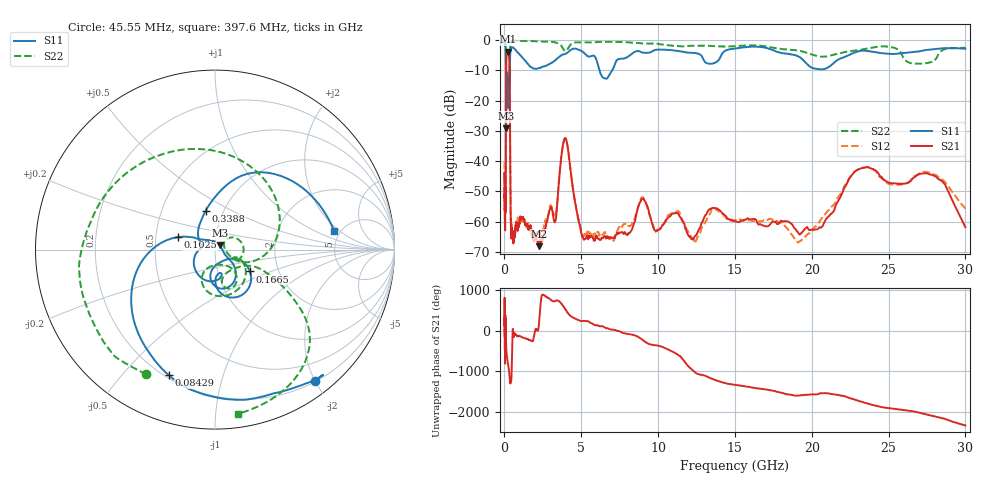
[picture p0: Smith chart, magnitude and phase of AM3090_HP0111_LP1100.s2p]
! Date/Time: Thu, Feb 28, 2019 2:01 PM
! Network Analyzer: Agilent Technologies E8364B Rev: A.07.50.67
! Sweep from 0.010 to 30.000 GHz, 1601 Points, Sweep Type: LOG
! Power Supply: 5.023 V, 0.002 A
# Hz S DB R 50
!freq MagS11 AngS11 MagS21 AngS21 MagS12 AngS12 MagS22 AngS22
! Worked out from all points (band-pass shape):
!   1601 points, 10 MHz to 30 GHz, reference 50 ohm
!   highest |S21| = -3.79 dB at 228.2 MHz (marker M1); lowest = -68.2 dB at 2.246 GHz (marker M2)
!   |S21| within 3 dB of the highest: 115.2 MHz to 321 MHz (205.8 MHz wide, 94.4 % of centre)
!   lowest |S11| = -29.1 dB at 109.9 MHz (marker M3), VSWR 1.07, Z = 52.6 + j2.44 ohm
!   |S11| at or under -10 dB: 100.6 MHz to 349.8 MHz (249.2 MHz wide, 111 % of centre); 6.184 GHz to 7.01 GHz (825.8 MHz wide, 12.5 % of centre)
!   |S22| runs from -25.4 to -0.1 dB; largest |S21 - S12| = 0.014
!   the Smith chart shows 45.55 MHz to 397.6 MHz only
!   S11 on the Smith chart (normalised r, x): 45.55 MHz: 0.21, -2.01; 84.29 MHz: 0.21, -0.68; 102.5 MHz: 0.65, +0.09; 166.5 MHz: 1.43, -0.37; 338.8 MHz: 0.82, +0.38; 397.6 MHz: 4.45, +1.66
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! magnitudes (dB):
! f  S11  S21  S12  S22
! 10 MHz  -0.2  -47.2  -40.4  -0.6
! 38.04 MHz  -0.5  -58.5  -59.6  -1.5
! 45.55 MHz  -0.7  -54.2  -54.9  -2.0
! 84.29 MHz  -2.5  -51.4  -53.1  -4.7
! 102.5 MHz  -13.2  -16.3  -16.3  -12.7
! 109.9 MHz  -29.1  -8.7  -8.7  -24.8
! 125.2 MHz  -13.1  -5.4  -5.4  -16.6
! 144.7 MHz  -21.9  -4.2  -4.2  -18.6
! 166.5 MHz  -12.8  -3.9  -3.8  -14.8
! 228.2 MHz  -17.4  -3.8  -3.8  -17.8
! 338.8 MHz  -13.0  -10.7  -10.7  -8.0
! 397.6 MHz  -3.5  -54.4  -55.0  -0.7
! 550.5 MHz  -2.5  -64.6  -66.6  -0.2
! 2.084 GHz  -9.5  -65.4  -63.8  -0.4
! 2.246 GHz  -9.2  -68.2  -64.3  -0.4
! 3.302 GHz  -6.7  -60.1  -58.2  -0.8
! 3.953 GHz  -4.6  -32.4  -32.4  -3.6
! 5.128 GHz  -4.0  -65.6  -64.5  -0.8
! 7.926 GHz  -5.8  -64.3  -61.2  -0.7
! 19.31 GHz  -6.0  -63.8  -66.3  -3.6
! 23.48 GHz  -3.5  -42.1  -42.1  -2.9
! 30 GHz  -2.8  -61.9  -55.7  -2.6
